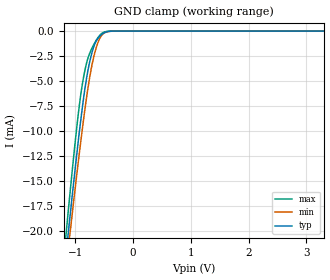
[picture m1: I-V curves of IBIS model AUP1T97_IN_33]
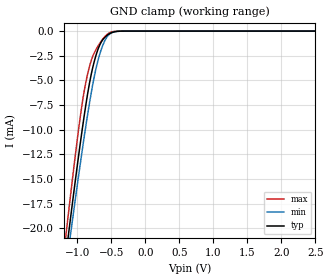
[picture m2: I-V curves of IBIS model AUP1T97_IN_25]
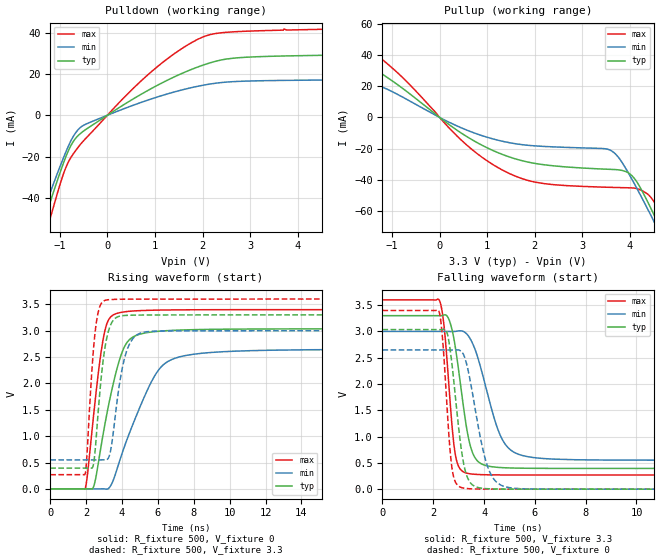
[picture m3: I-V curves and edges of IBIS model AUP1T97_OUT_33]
| TEXAS INSTRUMENTS INCORPORATED
| Standard Linear and Logic Group
| IBIS Model of SN74AUP1T97
| SINGLE-SUPPLY VOLTAGE TRANSLATOR
| This file contains package information for the following:
|  SOT 6-pin (DBV) package as [Component] AUP1T97_DBV
|  SOT 6-pin (DCK) package as [Component] AUP1T97_DCK
|  DSBGA 6-pin (YEP_YZP) package as [Component] AUP1T97_YEP_YZP
| This device can be powered at the following Vccs:
|  3.3 volt Vcc
|  2.5 volt Vcc
| This file provides unique models under the [Model Selector] for each Vcc.
| For operation at a specific Vcc, select the appropriate model after each
| [Model Selector] keyword.
[IBIS Ver]   3.2
[Comment char]  |_char
[File Name]   sn74aup1t97.ibs
[File Rev]   1.1 | x_die
[Date]   July 20, 2004
[Source]   Data created from TI-SPICE simulations at TI-SLL.
[Notes]   The following is an IBIS list for the AUP1T97.
   Please contact sllibis@ti.com with questions and
   comments concerning SLL IBIS models.
   - FILE REV HISTORY
   - 1.1 Release IBIS file on 10/01/04
   - Non-monotonic data in pullup due to special output circuit.
   - Power clamp data deleted as there is no power-clamp diode.
   - YEP and YZP packages are package preview only at this date.
[Disclaimer] Property of Texas Instruments Incorporated.  Unauthorized
   reproduction and/or distribution is strictly prohibited.
   This product is protected under copyright law.
   Created  2004, (C) Copyright  2004, Texas Instruments
   Incorporated, All Rights Reserved
   UNLESS THERE IS A SIGNED, WRITTEN AGREEMENT TO THE
   CONTRARY, TEXAS INSTRUMENTS (TI) IS PROVIDING THE IBIS
   MODELS  AND WITHOUT ANY WARRANTY, EXPRESSED OR
   IMPLIED.  TI assumes no liability for:
   1) the accuracy of the IBIS models provided to your
   company;
   2) the proper functioning of these IBIS Models in your
   design or for any resulting applications; or
   3) infringement of patents, copyrights or intellectual
   property rights resulting from your use of these IBIS
   models.
   TI provides IBIS Models as a service to our customers.
   You and your company shall not distribute, sell or give
   these models to anyone else without prior written
   permission from TI.
   TI reserves the right to make changes to our products or
   to discontinue any semiconductor product or service
   without notice, and advises our customers to obtain the
   latest version of relevant information to verify, before
   placing orders, that the information being relied on is
   current.
   Please be aware that your receipt and use of the IBIS
   information provided shall serve as acceptance of these
   terms and conditions.  If you do not accept these terms,
   you should return or destroy the IBIS models and any
   other accompanying information immediately.
| Component AUP1T97_DBV 6-pin SOT
[Component]   AUP1T97_DBV
[Manufacturer]   Texas Instruments, Inc.
[Package]
|   typ   min   max
R_pkg   2.500e-02   1.900e-02   3.700e-02
L_pkg   1.524e-09   1.260e-09   1.751e-09
C_pkg   2.450e-13   1.980e-13   2.640e-13
[Pin]   signal_name   model_name   R_pin   L_pin   C_pin
1   B   AUP1T97_IN   2.100e-02   1.405e-09   2.460e-13
2   GND   GND   3.700e-02   1.751e-09   2.630e-13
3   A   AUP1T97_IN   2.600e-02   1.493e-09   2.470e-13
4   Y   AUP1T97_OUT   1.900e-02   1.620e-09   2.640e-13
5   VCC   POWER   2.400e-02   1.260e-09   1.980e-13
6   C   AUP1T97_IN   2.100e-02   1.617e-09   2.500e-13
| Component AUP1T97_DCK 6-pin SOT
[Component]   AUP1T97_DCK
[Manufacturer]   Texas Instruments, Inc.
[Package]
|   typ   min   max
R_pkg   1.400e-02   1.100e-02   2.100e-02
L_pkg   9.480e-10   7.840e-10   1.103e-09
C_pkg   1.910e-13   1.670e-13   2.050e-13
[Pin]   signal_name   model_name   R_pin   L_pin   C_pin
1   B   AUP1T97_IN   1.300e-02   9.840e-10   1.960e-13
2   GND   GND   2.100e-02   1.103e-09   2.050e-13
3   A   AUP1T97_IN   1.100e-02   9.980e-10   1.970e-13
4   Y   AUP1T97_OUT   1.300e-02   9.040e-10   1.900e-13
5   VCC   POWER   1.500e-02   7.840e-10   1.670e-13
6   C   AUP1T97_IN   1.200e-02   9.160e-10   1.950e-13
| Component AUP1T97_YEP_YZP 6-pin DSBGA
[Component]   AUP1T97_YEP_YZP
[Manufacturer]   Texas Instruments, Inc.
[Package]
|   typ   min   max
R_pkg   1.000e-03   1.000e-03   2.100e-02
L_pkg   2.450e-11   2.400e-11   1.103e-09
C_pkg   5.600e-14   0.000e+00   2.050e-13
[Pin]   signal_name   model_name   R_pin   L_pin   C_pin
1   B   AUP1T97_IN   1.000e-03   2.500e-11   6.400e-14
2   GND   GND   1.000e-03   2.400e-11   6.700e-14
3   A   AUP1T97_IN   1.000e-03   2.500e-11   6.400e-14
4   Y   AUP1T97_OUT   1.000e-03   2.500e-11   6.400e-14
5   VCC   POWER   1.000e-03   2.400e-11   6.700e-14
6   NA/B   AUP1T97_IN   1.000e-03   2.500e-11   6.400e-14
| Model AUP1T97_IN
[Model Selector]   AUP1T97_IN
AUP1T97_IN_33   3.3 volt Vcc
AUP1T97_IN_25   2.5 volt Vcc
| Model AUP1T97_OUT
[Model Selector]   AUP1T97_OUT
AUP1T97_OUT_33   3.3 volt Vcc
AUP1T97_OUT_25   2.5 volt Vcc
| Models and submodels in the file (4): AUP1T97_IN_33 (Input), AUP1T97_IN_25 (Input), AUP1T97_OUT_33 (Output), AUP1T97_OUT_25 (Output)
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[Model]   AUP1T97_IN_33
Model_type  Input
Vinl=0.9
Vinh=2.1
| variable   typ   min   max
C_comp   1.42pF   1.16pF   1.79pF
[Temperature Range]   40   100   -40
| Ambient temperature   25   85   -40
[Voltage range]   3.3   3   3.6
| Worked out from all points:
|   GND clamp passes 1 mA (typ) near -0.64 V on its own axis
[GND Clamp]
| AUP1T97_IN_33
|   Voltage   I(typ)   I(min)   I(max)
-3.6V     -171.6mA   -163.5mA   -181.1mA
-1.16V    -22.22mA   -23.69mA   -20.18mA
-1.11V    -19.45mA   -21.09mA   -17.19mA
-1.085V   -18.08mA   -19.81mA   -15.71mA
-940mV    -10.5mA    -12.6mA    -7.822mA
-890mV    -8.117mA   -10.26mA   -5.698mA
-835mV    -5.768mA   -7.825mA   -3.925mA
-755mV    -3.153mA   -4.717mA   -2.255mA
-675mV    -1.463mA   -2.419mA   -1.277mA
-595mV    -617.7uA   -945.8uA   -546.7uA
-515mV    -215.4uA   -248.8uA   -134.4uA
3.3V      132.2pA    540.4pA    36.28pA
[Model]   AUP1T97_IN_25
Model_type  Input
Vinl=0.7
Vinh=1.6
| variable   typ   min   max
C_comp   1.46pF   1.21pF   1.77pF
[Temperature Range]   40   100   -40
| Ambient temperature   25   85   -40
[Voltage range]   2.5   2.3   2.7
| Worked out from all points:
|   GND clamp passes 1 mA (typ) near -0.64 V on its own axis
[GND Clamp]
| AUP1T97_IN_25
|   Voltage   I(typ)   I(min)   I(max)
-3.6V     -171.6mA   -163.5mA   -181.1mA
-1.165V   -22.5mA    -23.95mA   -20.48mA
-1.115V   -19.72mA   -21.35mA   -17.49mA
-1.09V    -18.36mA   -20.06mA   -16.01mA
-945mV    -10.75mA   -12.84mA   -8.061mA
-890mV    -8.117mA   -10.26mA   -5.698mA
-835mV    -5.768mA   -7.825mA   -3.925mA
-760mV    -3.287mA   -4.89mA    -2.329mA
-675mV    -1.463mA   -2.419mA   -1.277mA
-595mV    -617.7uA   -945.8uA   -546.7uA
-520mV    -233.1uA   -272.6uA   -149.9uA
2.5V      104.3pA    491.9pA    26.71pA
[Model]   AUP1T97_OUT_33
Model_type  Output
Vref =   0
Rref =   1E6
Cref =   30p
Vmeas =   1.65
| variable   typ   min   max
C_comp   2.73pF   1.81pF   4.12pF
| C_pullup   3.12pF   1.81pF   4.12pF
| C_pulldown   2.33pF   2.13pF   2.90pF
[Temperature Range]   40   100   -40
| Ambient temperature   25   85   -40
[Voltage range]   3.3   3   3.6
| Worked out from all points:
|   slope of the pulldown table from 0 to 0.495 V, typ, clamps not added: 68.4 ohm
|   slope of the pullup table from 0 to 0.495 V, typ, clamps not added: 45.8 ohm
|   rising waveform, R_fixture 500, V_fixture 0: 20-80 % time 1.11ns typ, 1.91ns min, 689ps max; typ from 0 V to 3.04 V
|   falling waveform, R_fixture 500, V_fixture 3.3: 20-80 % time 523ps typ, 876ps min, 333ps max; typ from 3.3 V to 0.394 V
|   rising waveform, R_fixture 500, V_fixture 3.3: 20-80 % time 506ps typ, 664ps min, 393ps max; typ from 0.394 V to 3.3 V
|   falling waveform, R_fixture 500, V_fixture 0: 20-80 % time 428ps typ, 642ps min, 284ps max; typ from 3.04 V to 0 V
[Pulldown]
| AUP1T97_OUT_33
|   Voltage   I(typ)   I(min)   I(max)
-3.6V     -218.7mA   -196.3mA   -248.6mA
-1.515V   -64.37mA   -57.31mA   -75.82mA
-1.39V    -55.35mA   -49.29mA   -65.41mA
-1.275V   -47.14mA   -42mA      -55.89mA
-870mV    -19.93mA   -17.62mA   -25.18mA
-720mV    -12.85mA   -10.38mA   -18.82mA
-545mV    -8.444mA   -5.509mA   -13.51mA
940mV     13.13mA    8.018mA    21.36mA
1.5V      19.56mA    11.86mA    31.27mA
2.045V    24.53mA    14.67mA    38.2mA
3.1V      28.27mA    16.63mA    40.81mA
7.2V      29.73mA    17.36mA    42.67mA
[Pullup]
| AUP1T97_OUT_33
|   Voltage   I(typ)   I(min)   I(max)
-3.6V     42.88mA    27.27mA    57.92mA
-2.465V   31.53mA    19.52mA    45.85mA
-1.53V    32.87mA    22.09mA    44.95mA
-755mV    18.1mA     12.64mA    24.89mA
555mV     -11.98mA   -7.942mA   -17.3mA
1.65V     -27.07mA   -17.13mA   -38.31mA
3.61V     -33.32mA   -21.39mA   -44.82mA
4.08V     -38.63mA   -41.77mA   -45.28mA
4.375V    -54.25mA   -58.9mA    -49.24mA
4.565V    -66.24mA   -70.37mA   -57.33mA
4.775V    -80.02mA   -83.29mA   -71.37mA
7.2V      -250.7mA   -240.9mA   -257mA
[Ramp]
| AUP1T97_OUT_33
| variable   typ   min   max
dV/dt_r   1.82/1.11E-09   1.59/1.92E-09   2.04/6.91E-10
dV/dt_f   1.75/5.30E-10   1.48/8.84E-10   2.01/3.35E-10
R_load = 500
[Rising Waveform]
| AUP1T97_OUT_33
R_fixture =   500
C_fixture =   0
L_fixture =   0
V_fixture =   0
V_fixture_min = 0
V_fixture_max = 0
|   Time   V(typ)   V(min)   V(max)
0s        24.73nV    82.54nV    2.123nV
1.95ns    -15.76uV   474.7nV    14.63mV
2.43ns    56.89mV    -19.15uV   1.444V
2.94ns    1.026V     2.126mV    2.823V
3.235ns   1.562V     4.791mV    3.196V
3.685ns   2.237V     336.5mV    3.325V
4.38ns    2.819V     1.03V      3.367V
5.74ns    2.979V     2.096V     3.389V
7.22ns    3.012V     2.505V     3.395V
29.99ns   3.035V     2.647V     3.399V
[Falling Waveform]
| AUP1T97_OUT_33
R_fixture =   500
C_fixture =   0
L_fixture =   0
V_fixture =   3.3
V_fixture_min = 3
V_fixture_max = 3.6
|   Time   V(typ)   V(min)   V(max)
0s        3.3V       3V         3.6V
2.245ns   3.299V     3V         3.587V
2.435ns   3.314V     3V         3.052V
2.64ns    3.198V     2.999V     1.808V
2.855ns   2.741V     3V         699.3mV
3.33ns    1.115V     2.946V     303.2mV
3.735ns   539.1mV    2.531V     279.8mV
4.68ns    410.4mV    980.9mV    270.6mV
5.705ns   397.6mV    618.9mV    269.5mV
29.99ns   394.1mV    550mV      269.3mV
[Rising Waveform]
| AUP1T97_OUT_33
R_fixture =   500
C_fixture =   0
L_fixture =   0
V_fixture =   3.3
V_fixture_min = 3
V_fixture_max = 3.6
|   Time   V(typ)   V(min)   V(max)
0s        394.1mV    550mV      269.3mV
1.945ns   394mV      550mV      289.5mV
2.355ns   407.4mV    550mV      2.417V
2.505ns   746mV      550mV      2.989V
2.745ns   1.765V     550.2mV    3.441V
3.065ns   2.714V     550mV      3.577V
3.365ns   3.11V      729.5mV    3.591V
4.185ns   3.289V     2.534V     3.598V
5.13ns    3.297V     2.965V     3.599V
29.99ns   3.3V       3V         3.6V
[Falling Waveform]
| AUP1T97_OUT_33
R_fixture =   500
C_fixture =   0
L_fixture =   0
V_fixture =   0
V_fixture_min = 0
V_fixture_max = 0
|   Time   V(typ)   V(min)   V(max)
0s        3.035V     2.647V     3.399V
2.22ns    3.035V     2.647V     3.387V
2.36ns    3.037V     2.647V     2.886V
2.53ns    2.99V      2.647V     1.659V
2.725ns   2.422V     2.647V     443.5mV
3.155ns   595.8mV    2.589V     24.03mV
3.46ns    121.7mV    2.047V     7.41mV
4.125ns   8.998mV    449.1mV    922.3uV
4.94ns    1.048mV    33.24mV    111.9uV
29.99ns   2.652nV    82.2nV     -13.61nV
